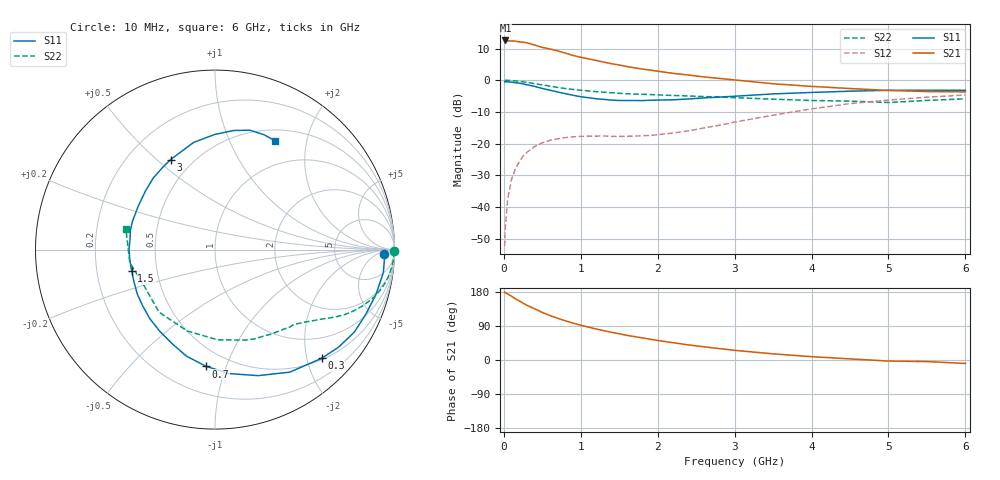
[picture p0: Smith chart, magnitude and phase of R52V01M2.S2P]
! SIEMENS Small Signal Semiconductors
! BFR183
! Si NPN RF Bipolar Junction Transistor in SOT23
! VCE = 2 V  IC = 1.2 mA
! Common Emitter S-Parameters:  May  1996
# GHz  S  MA  R  50
!  f  S11  S21  S12  S22
! GHz  MAG  ANG  MAG  ANG  MAG  ANG  MAG  ANG
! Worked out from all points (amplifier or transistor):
!   36 points, 10 MHz to 6 GHz, reference 50 ohm
!   highest |S21| = 12.6 dB at 20 MHz (marker M1)
!   |S21| within 3 dB of that: start of sweep to 650.5 MHz
!   unconditionally stable (mu >= 1): 1.568 GHz to 2.942 GHz
!   at 250 MHz: K = 0.17, MSG = 18.0 dB, |S12| = -24.0 dB
!   at 1.4 GHz: K = 0.91, MSG = 11.5 dB, |S12| = -17.7 dB
!   at 6 GHz: K = 0.95, MSG = 0.5 dB, |S12| = -4.7 dB
!   S11 on the Smith chart (normalised r, x): 10 MHz: 28, -13; 300 MHz: 0.53, -2.28; 700 MHz: 0.38, -0.85; 1.5 GHz: 0.36, -0.11; 3 GHz: 0.38, +0.55; 6 GHz: 0.64, +1.50
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0.01  0.9434 -1.6  4.172 179.2  0.0024 86.9  0.9994 -0.6
0.02  0.9456 -3.4  4.249 177.4  0.0049 87.2  0.996 -1.2
0.05  0.9465 -7.8  4.191 174.1  0.0134 85.4  0.9957 -3.0
0.1  0.9311 -15.5  4.177 168.3  0.0271 81.1  0.9892 -5.9
0.15  0.9142 -23.2  4.139 161.5  0.0398 76.6  0.9778 -8.9
0.3  0.8488 -45.5  3.894 144.3  0.0728 64.0  0.9266 -16.5
0.4  0.7999 -58.6  3.599 135.2  0.0897 56.9  0.8837 -20.6
0.5  0.7422 -71.1  3.301 125.5  0.1027 51.2  0.8443 -23.9
0.6  0.6955 -83.4  3.118 117.3  0.1127 46.3  0.8058 -26.8
0.7  0.6527 -94.3  2.904 110.1  0.1192 42.5  0.7704 -29.1
0.8  0.6145 -105.0  2.678 103.3  0.1244 39.1  0.7393 -31.1
0.9  0.5781 -113.9  2.462 97.3  0.128 36.7  0.7158 -32.6
1.1  0.5293 -133.2  2.176 86.8  0.131 33.5  0.6775 -35.7
1.3  0.4987 -150.3  1.936 77.3  0.1316 32.3  0.6468 -38.5
1.5  0.4791 -165.7  1.744 69.3  0.13 33.8  0.6225 -41.3
1.9  0.4835 167.0  1.447 54.8  0.1345 39.9  0.5943 -47.4
2.2  0.4912 150.7  1.284 45.6  0.1467 46.1  0.5751 -52.5
3  0.559 116.3  1.012 25.5  0.2183 54.6  0.5311 -71.7
3.5  0.609 101.3  0.88 16.2  0.2805 52.6  0.5028 -88.3
4.5  0.6718 81.1  0.74 2.9  0.4282 39.9  0.4678 -131.7
5.5  0.6959 66.8  0.663 -4.2  0.5403 23.5  0.4802 -171.3
6  0.6924 61.0  0.655 -9.1  0.5851 13.7  0.509 167.2
